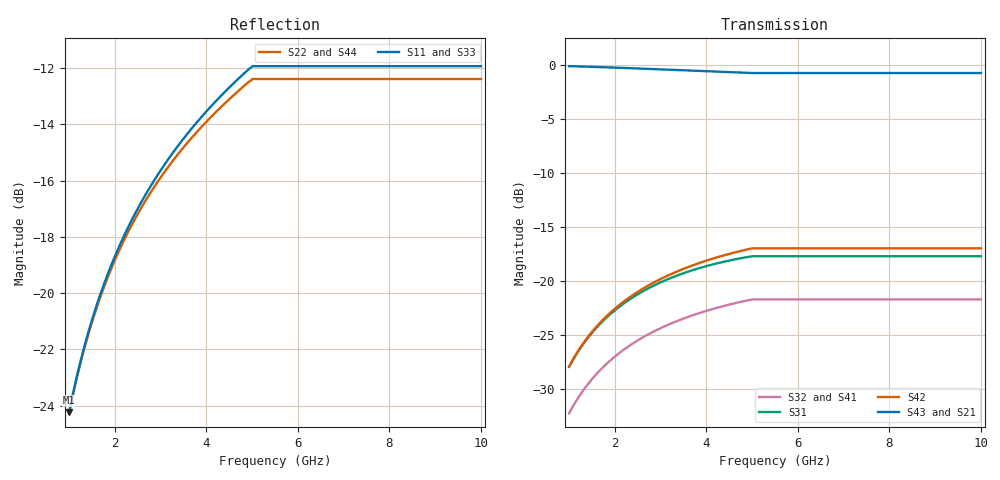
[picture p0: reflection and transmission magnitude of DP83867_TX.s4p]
! Created Fri May 12 13:39:06 2017
# hz S db R 50
! 4 Port Network Data from SP1.SP block
! freq  dbS11  angS11  dbS12  angS12  dbS13  angS13  dbS14  angS14
!  dbS21  angS21  dbS22  angS22  dbS23  angS23  dbS24  angS24
!  dbS31  angS31  dbS32  angS32  dbS33  angS33  dbS34  angS34
!  dbS41  angS41  dbS42  angS42  dbS43  angS43  dbS44  angS44
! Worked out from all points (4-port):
!   101 points, 1 GHz to 10 GHz, reference 50 ohm
!   strongest paths, dB at 1 GHz, 1.778 GHz, 3.162 GHz, 5.623 GHz, 10 GHz:
!     S43: -0.1, -0.2, -0.4, -0.7, -0.7
!     S21: -0.1, -0.2, -0.5, -0.8, -0.8
!     S42: -28.0, -23.5, -19.5, -17.0, -17.0
!     S31: -28.0, -23.6, -19.8, -17.7, -17.7
!     S32: -32.3, -27.9, -24.1, -21.7, -21.7
!     S41: -32.3, -27.9, -24.1, -21.7, -21.7
!   lowest |S11| = -24.2 dB at 1 GHz (marker M1), VSWR 1.13, Z = 51.7 + j6.03 ohm
!   |S11| at or under -10 dB: start of sweep to end of sweep
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1e9  -24.23 71.2  -0.09 -8.8  -28.00 73.0  -32.30 -112.1
     -0.09 -8.8  -24.27 78.9  -32.30 -111.7  -27.96 75.4
     -28.00 73.0  -32.30 -111.7  -24.60 72.6  -0.08 -8.3
     -32.30 -112.1  -27.96 75.4  -0.08 -8.3  -24.63 79.4
1.28825e9  -22.17 66.9  -0.13 -11.3  -25.99 68.9  -30.30 -117.7
           -0.13 -11.3  -22.23 76.8  -30.30 -117.2  -25.93 71.9
           -25.99 68.9  -30.30 -117.2  -22.53 68.8  -0.12 -10.6
           -30.30 -117.7  -25.93 71.9  -0.12 -10.6  -22.57 77.5
1.62181e9  -20.33 62.1  -0.18 -14.0  -24.25 64.2  -28.55 -124.0
           -0.18 -14.0  -20.42 74.6  -28.55 -123.4  -24.15 67.9
           -24.25 64.2  -28.55 -123.4  -20.68 64.4  -0.16 -13.3
           -28.55 -124.0  -24.15 67.9  -0.16 -13.3  -20.75 75.4
2.454709e9  -17.13 50.6  -0.33 -20.7  -21.37 53.7  -25.65 -138.6
            -0.33 -20.7  -17.32 69.8  -25.65 -137.7  -21.16 59.1
            -21.37 53.7  -25.65 -137.7  -17.45 54.0  -0.29 -19.6
            -25.65 -138.6  -21.16 59.1  -0.29 -19.6  -17.59 70.8
3.548134e9  -14.41 37.0  -0.53 -29.1  -19.23 41.7  -23.44 -155.8
            -0.53 -29.1  -14.73 64.8  -23.43 -154.5  -18.81 49.0
            -19.23 41.7  -23.43 -154.5  -14.69 41.5  -0.47 -27.7
            -23.44 -155.8  -18.81 49.0  -0.47 -27.7  -14.92 66.0
4.897788e9  -12.08 21.7  -0.79 -39.1  -17.80 29.1  -21.83 -174.8
            -0.79 -39.1  -12.53 60.2  -21.82 -172.9  -17.09 38.1
            -17.80 29.1  -21.82 -172.9  -12.33 27.4  -0.70 -37.2
            -21.83 -174.8  -17.09 38.1  -0.70 -37.2  -12.67 61.2
1e10  -11.93 20.6  -0.80 -39.8  -17.72 28.2  -21.74 -176.1
      -0.80 -39.8  -12.39 59.9  -21.73 -174.3  -16.99 37.4
      -17.72 28.2  -21.73 -174.3  -12.18 26.3  -0.72 -37.9
      -21.74 -176.1  -16.99 37.4  -0.72 -37.9  -12.52 60.9
